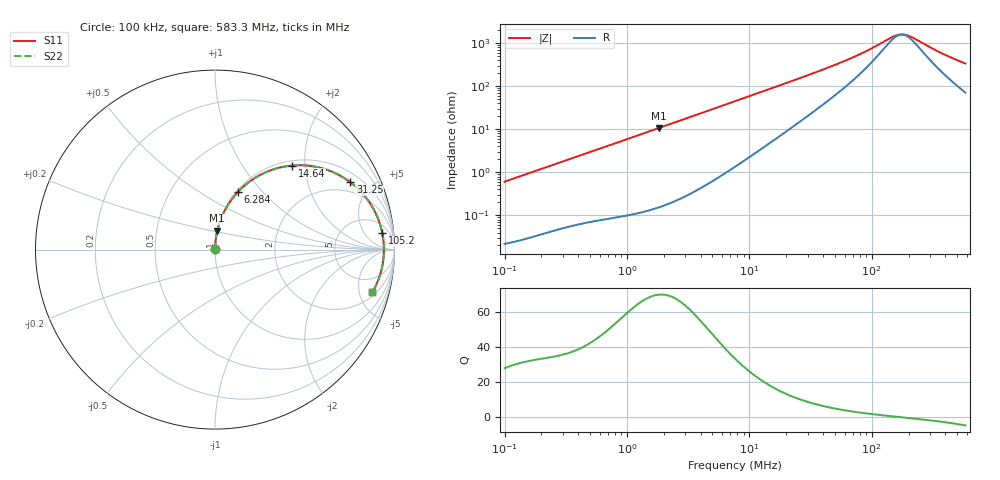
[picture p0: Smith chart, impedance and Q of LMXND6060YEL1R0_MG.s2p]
! LMXND6060YEL1R0_MG  S-PARAMETER MODEL  ( General Type )
! Model Generated by TAIYO YUDEN Corporation (http://www.ty-top.com)
! Version 1.0
! TAIYO YUDEN Control No. 191025NI43SB-FBB
! Copyright(c) 2019 TAIYO YUDEN CO.,LTD. All Rights Reserved.
! Product Description (link to TY-COMPAS)
! https://ds.yuden.co.jp/TYCOMPAS/or/detail?pn=LMXND6060YEL1R0NMG&u=M
! Products Name : Inductors
! Characteristics :
!  Inductance : 1.0 uH , SRF(min) : 110 MHz , DC Resistance(max) : 0.0182 Ohm
!  Rated Current : Saturation :9800 mA , Temp Rise : 4500 mA
!  Case Size : 6.0 x 6.0 / 0.236 x 0.236 [mm/inch] , Thickness : 4.5 / 0.177 [mm/inch]
!  (Conditions: Temperature = 25 degC , DC Bias Current/Voltage = 0A / 0V)
! External Node Assignments :
!  1  o---GGG---o  2
! GND o---------o GND
! Frequency Range : 0.1MHz  -  583.332491MHz  [ 402 STEP ]
# MHz S RI R 50
! Freq[MHz].  S11 Real  S11 Imag  S21 Real  S21 Imag  S12 Real  S12 Imag  S22 Real  S22 Imag
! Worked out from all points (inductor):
!   401 points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, 100 kHz to 583.3 MHz, reference 50 ohm
!   read as one part in series: L = 965 nH near 104.4 kHz
!   highest Q = 69.8 at 1.826 MHz (marker M1), where L = 936 nH
!   self-resonance near 176.5 MHz
!   S11 on the Smith chart (normalised r, x): 100 kHz: 1.00, +0.01; 6.284 MHz: 1.02, +0.74; 14.64 MHz: 1.10, +1.73; 31.25 MHz: 1.44, +3.74; 105.2 MHz: 9, +14; 583.3 MHz: 2.42, -6.60
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0.1  0.000254 0.00607  0.9997 -0.00607  0.9997 -0.00607  0.000254 0.00607
0.427357  0.00129 0.0254  0.9987 -0.0254  0.9987 -0.0254  0.00129 0.0254
0.953099  0.0041 0.0559  0.9959 -0.0559  0.9959 -0.0559  0.0041 0.0559
1.826341  0.0129 0.1058  0.9871 -0.1058  0.9871 -0.1058  0.0129 0.1058
3.734823  0.0493 0.2079  0.9507 -0.2079  0.9507 -0.2079  0.0493 0.2079
6.283838  0.1263 0.3197  0.8737 -0.3197  0.8737 -0.3197  0.1263 0.3197
7.637621  0.1752 0.3655  0.8248 -0.3655  0.8248 -0.3655  0.1752 0.3655
10.34583  0.2785 0.429  0.7215 -0.429  0.7215 -0.429  0.2785 0.429
14.63531  0.4313 0.4685  0.5687 -0.4685  0.5687 -0.4685  0.4313 0.4685
20.70325  0.5946 0.4536  0.4054 -0.4536  0.4054 -0.4536  0.5946 0.4536
31.255  0.7549 0.3748  0.2451 -0.3748  0.2451 -0.3748  0.7549 0.3748
32.63992  0.7683 0.3642  0.2317 -0.3642  0.2317 -0.3642  0.7683 0.3642
44.21362  0.8437 0.2866  0.1563 -0.2866  0.1563 -0.2866  0.8437 0.2866
62.54502  0.8962 0.2007  0.1038 -0.2007  0.1038 -0.2007  0.8962 0.2007
82.90582  0.9203 0.1386  0.0797 -0.1386  0.0797 -0.1386  0.9203 0.1386
105.232  0.9322 0.0915  0.0678 -0.0915  0.0678 -0.0915  0.9322 0.0915
139.489  0.9394 0.0405  0.0606 -0.0405  0.0606 -0.0405  0.9394 0.0405
155.4583  0.9407 0.0217  0.0593 -0.0217  0.0593 -0.0217  0.9407 0.0217
169.5404  0.9411 0.00686  0.0589 -0.00686  0.0589 -0.00686  0.9411 0.00686
197.3225  0.9408 -0.0191  0.0592 0.0191  0.0592 0.0191  0.9408 -0.0191
370.0033  0.9213 -0.1355  0.0787 0.1355  0.0787 0.1355  0.9213 -0.1355
583.3325  0.876 -0.2388  0.124 0.2388  0.124 0.2388  0.876 -0.2388
